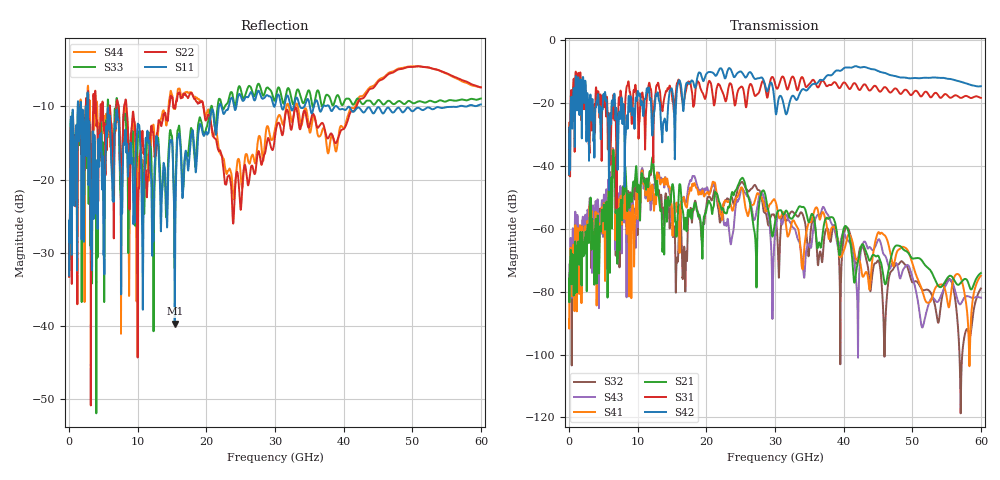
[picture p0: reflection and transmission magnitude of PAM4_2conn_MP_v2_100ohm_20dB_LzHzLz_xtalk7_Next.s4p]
! Info: Touchstone file created by Circ.  Input file=FAB50GbE_2conn_Midplane_Examax_Topo2_v2_100ohm_20dB_LzHzLz.circ
# Hz S RI R 50
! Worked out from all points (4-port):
!   6000 points, 10 MHz to 60 GHz, reference 50 ohm
!   strongest paths, dB at 10 MHz, 15.01 GHz, 30.01 GHz, 45.01 GHz, 60 GHz:
!     S42: -42.6, -15.7, -21.2, -9.7, -14.6
!     S31: -42.9, -18.0, -13.7, -15.6, -18.3
!     S21: -75.8, -46.2, -57.9, -68.5, -74.0
!     S41: -88.9, -57.0, -50.9, -61.2, -74.9
!     S43: -77.4, -55.4, -61.7, -63.5, -81.9
!     S32: -81.8, -56.0, -56.4, -70.0, -79.0
!   lowest |S11| = -39.7 dB at 15.4 GHz (marker M1), VSWR 1.02, Z = 49 - j0.352 ohm
!   |S11| at or under -10 dB: start of sweep to 1.262 GHz; 2.763 GHz to 21.84 GHz (19.08 GHz wide, 155 % of centre); 39.01 GHz to 56.78 GHz (17.78 GHz wide, 37.1 % of centre)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
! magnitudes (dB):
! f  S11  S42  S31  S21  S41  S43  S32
! 10 MHz  -33.1  -42.6  -42.9  -75.8  -88.9  -77.4  -81.8
! 1.16 GHz  -32.4  -22.3  -19.2  -76.1  -69.0  -60.5  -68.4
! 6.38 GHz  -22.8  -20.4  -23.2  -36.3  -34.7  -34.3  -36.1
! 15.4 GHz  -39.7  -36.8  -19.5  -55.3  -53.1  -52.0  -60.9
! 25.19 GHz  -9.1  -10.2  -14.7  -43.8  -46.8  -47.3  -45.0
! 27.16 GHz  -9.0  -12.3  -17.7  -64.0  -50.4  -56.2  -46.2
! 60 GHz  -9.7  -14.6  -18.3  -74.0  -74.9  -81.9  -79.0
